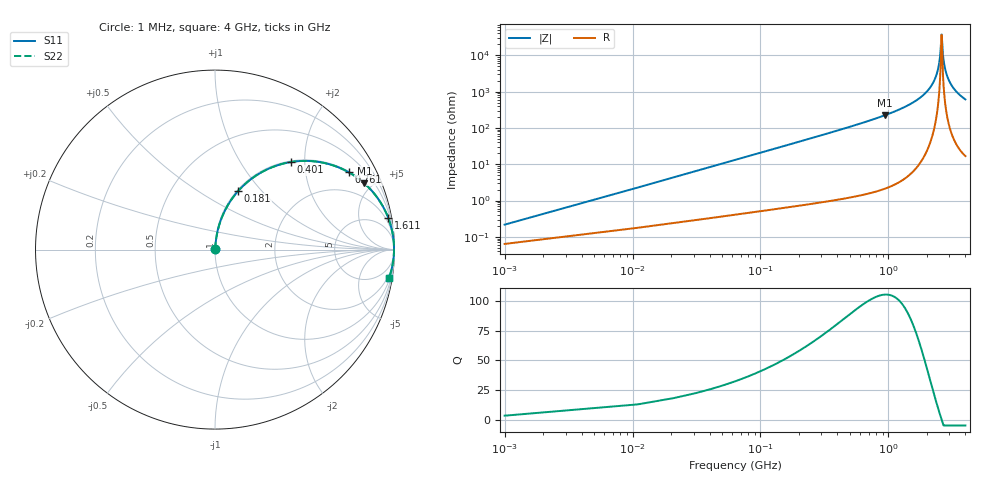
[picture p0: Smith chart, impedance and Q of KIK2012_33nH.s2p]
!version-2
!date-01.2022
!Series
# MHz S RI R 50
!Freq ReS11 ImS11 ReS21 ImS21 ReS12 ImS12 ReS22 ImS22
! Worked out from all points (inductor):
!   401 points, 1 MHz to 4 GHz, reference 50 ohm
!   read as one part in series: L = 33 nH near 21 MHz
!   highest Q = 106 at 941 MHz (marker M1), where L = 37.9 nH
!   self-resonance near 2.601 GHz
!   S11 on the Smith chart (normalised r, x): 1 MHz: 1.00, +0.00; 181 MHz: 1.01, +0.75; 401 MHz: 1.02, +1.70; 761 MHz: 1.03, +3.45; 1.611 GHz: 1, +11; 4 GHz: 1, -12
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1  0.000643 0.00207  0.9994 -0.00207  0.9994 -0.00207  0.000643 0.00207
31  0.00696 0.0637  0.993 -0.0637  0.993 -0.0637  0.00696 0.0637
51  0.0146 0.1039  0.9854 -0.1039  0.9854 -0.1039  0.0146 0.1039
101  0.0466 0.1989  0.9534 -0.1989  0.9534 -0.1989  0.0466 0.1989
181  0.129 0.3262  0.871 -0.3262  0.871 -0.3262  0.129 0.3262
401  0.4214 0.4876  0.5786 -0.4876  0.5786 -0.4876  0.4214 0.4876
671  0.6877 0.4584  0.3123 -0.4584  0.3123 -0.4584  0.6877 0.4584
761  0.7464 0.4302  0.2536 -0.4302  0.2536 -0.4302  0.7464 0.4302
941  0.8319 0.3692  0.1681 -0.3692  0.1681 -0.3692  0.8319 0.3692
1341  0.9324 0.2459  0.0676 -0.2459  0.0676 -0.2459  0.9324 0.2459
1611  0.9647 0.178  0.0353 -0.178  0.0353 -0.178  0.9647 0.178
2001  0.9881 0.0975  0.0119 -0.0975  0.0119 -0.0975  0.9881 0.0975
2251  0.9947 0.054  0.00528 -0.054  0.00528 -0.054  0.9947 0.054
2421  0.9968 0.0272  0.00317 -0.0272  0.00317 -0.0272  0.9968 0.0272
2521  0.9973 0.0123  0.00265 -0.0123  0.00265 -0.0123  0.9973 0.0123
2601  0.9974 0.000761  0.00256 -0.000761  0.00256 -0.000761  0.9974 0.000761
2621  0.9974 -0.00206  0.00258 0.00206  0.00258 0.00206  0.9974 -0.00206
2671  0.9973 -0.00902  0.0027 0.00902  0.0027 0.00902  0.9973 -0.00902
2751  0.9969 -0.0199  0.00309 0.0199  0.00309 0.0199  0.9969 -0.0199
2881  0.9958 -0.0369  0.00419 0.0369  0.00419 0.0369  0.9958 -0.0369
3341  0.9881 -0.0914  0.0119 0.0914  0.0119 0.0914  0.9881 -0.0914
4000  0.9699 -0.1577  0.0301 0.1577  0.0301 0.1577  0.9699 -0.1577
